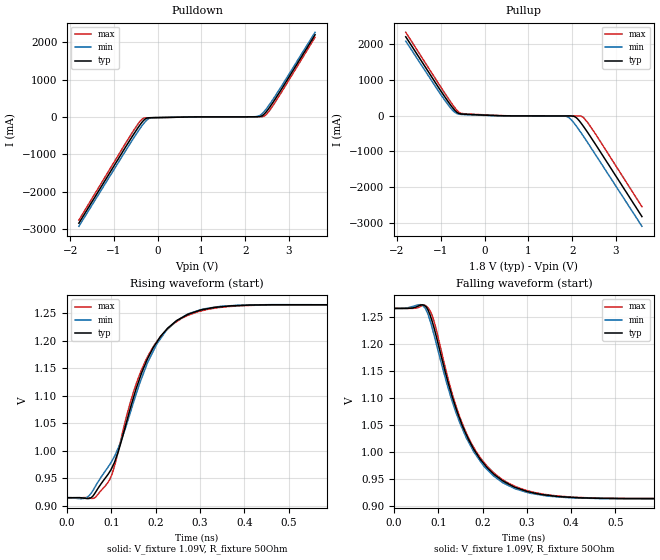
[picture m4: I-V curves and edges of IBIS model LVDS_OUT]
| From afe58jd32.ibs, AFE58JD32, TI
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|   Model
[Model]   LVDS_OUT
Model_type   Output
Polarity   Non-Inverting
Vmeas = 1.09
Vref = 1.09
Cref = 1pF
Rref = 50
|   typ   min   max
C_comp   1.633pF   1.601pF   1.676pF
[Voltage Range]   1.8   1.7   1.9
[Temperature Range]   25   85   -40
[Pullup Reference]   1.8   1.7   1.9
[Pulldown Reference]   -0   -0   -0
[Power Clamp Reference]   1.8   1.7   1.9
[GND Clamp Reference]   -0   -0   -0
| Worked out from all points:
|   slope of the pulldown table from 0 to 0.27 V, typ, clamps not added: 48.3 ohm
|   slope of the pullup table from 0 to 0.27 V, typ, clamps not added: 21.8 ohm
|   falling waveform, V_fixture 1.09V, R_fixture 50Ohm: 20-80 % time 95.9ps typ, 96.6ps min, 95.3ps max; typ from 1.26 V to 0.915 V
|   rising waveform, V_fixture 1.09V, R_fixture 50Ohm: 20-80 % time 91.1ps typ, 99.6ps min, 88.8ps max; typ from 0.915 V to 1.26 V
[Pulldown]
|   Voltage   I(typ)   I(min)   I(max)
-1.8V     -2.839A    -2.923A    -2.756A
-725.4mV  -787.4mA   -888mA     -685.4mA
-450mV    -286.1mA   -385.5mA   -185.8mA
-352.8mV  -132mA     -223.6mA   -52.86mA
-261mV    -36.37mA   -94.8mA    -21.51mA
-136.8mV  -17.39mA   -19.41mA   -18.62mA
2.201V    6.074mA    8.035mA    5.377mA
2.326V    12.01mA    35.74mA    6.45mA
2.434V    79.63mA    148.1mA    24.94mA
2.547V    243.5mA    323.5mA    161.9mA
2.671V    457.9mA    539mA      374.7mA
3.595V    2.201A     2.267A     2.134A
[Pullup]
|   Voltage   I(typ)   I(min)   I(max)
-1.8V     2.213A     2.091A     2.339A
-909mV    530.1mA    433.5mA    632.2mA
-703.8mV  185.9mA    121.8mA    264.1mA
-633.6mV  98.53mA    61.35mA    155.1mA
-552.6mV  51.69mA    37.63mA    72.38mA
457.2mV   -2.337mA   -3.799mA   98.8uA
1.818V    -6.916mA   -9.784mA   -6.415mA
1.926V    -7.162mA   -53.86mA   -6.578mA
2.099V    -59.54mA   -296.6mA   -6.852mA
2.25V     -284.2mA   -562.4mA   -42.07mA
2.363V    -485.5mA   -771.3mA   -205.4mA
3.595V    -2.828A    -3.101A    -2.552A
[Ramp]
R_load = 50
|   typ   min   max
dV/dt_r   0.210398/9.11245e-11   0.210118/9.96495e-11   0.210509/8.88293e-11
dV/dt_f   0.210379/9.59061e-11   0.210151/9.66127e-11   0.21051/9.53595e-11
[Falling Waveform]
V_fixture = 1.09V
V_fixture_min = 1.09V
V_fixture_max = 1.09V
R_fixture = 50Ohm
C_fixture = 0F
|   Time   V(typ)   V(min)   V(max)
0s        1.265V     1.265V     1.265V
60.41ps   1.271V     1.272V     1.269V
79.07ps   1.258V     1.249V     1.264V
91.43ps   1.227V     1.214V     1.239V
129.6ps   1.108V     1.099V     1.113V
177.2ps   1.01V      1.005V     1.013V
227.5ps   958mV      954.7mV    960.6mV
306ps     926.7mV    924.6mV    928.2mV
534ps     914.6mV    914.4mV    914.7mV
1.9ns     914.6mV    914.7mV    914.5mV
[Rising Waveform]
V_fixture = 1.09V
V_fixture_min = 1.09V
V_fixture_max = 1.09V
R_fixture = 50Ohm
C_fixture = 0F
|   Time   V(typ)   V(min)   V(max)
0s        914.6mV    914.9mV    914.5mV
49.31ps   913.2mV    917.9mV    914.2mV
91.43ps   955.9mV    968.9mV    941.3mV
115.1ps   997.1mV    1.004V     998mV
150.7ps   1.099V     1.09V      1.109V
186.1ps   1.174V     1.167V     1.177V
246.2ps   1.236V     1.236V     1.234V
306ps     1.256V     1.257V     1.255V
477.7ps   1.265V     1.265V     1.265V
1.9ns     1.265V     1.265V     1.265V
